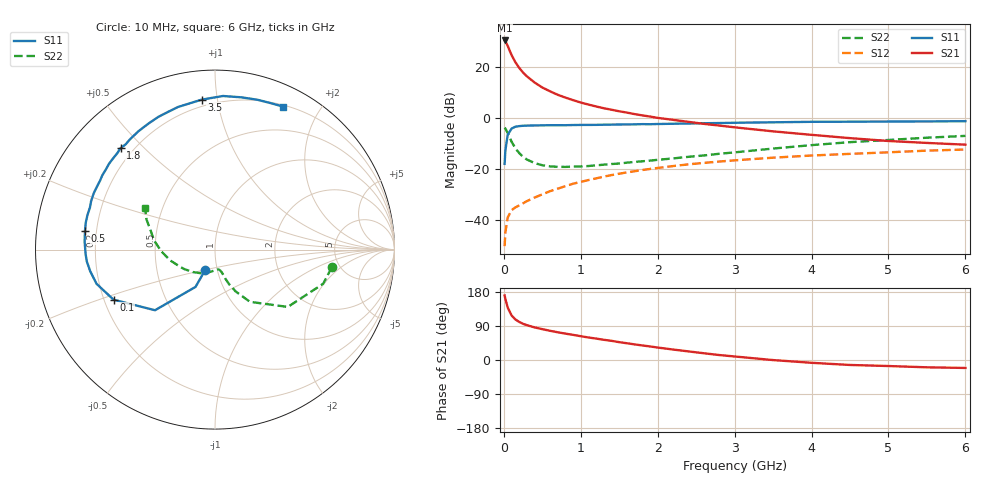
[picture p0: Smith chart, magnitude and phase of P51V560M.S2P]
! SIEMENS Small Signal Semiconductors
! BFP183
! Si NPN RF Bipolar Junction Transistor in SOT143
! VCE = 1.5 V  IC = 60 mA
! Common Emitter S-Parameters:  March  1996
# GHz  S  MA  R  50
!  f  S11  S21  S12  S22
! GHz  MAG  ANG  MAG  ANG  MAG  ANG  MAG  ANG
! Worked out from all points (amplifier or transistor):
!   36 points, 10 MHz to 6 GHz, reference 50 ohm
!   highest |S21| = 30.6 dB at 10 MHz (marker M1)
!   |S21| within 3 dB of that: start of sweep to 62.21 MHz
!   unconditionally stable (mu >= 1): start of sweep to 38.8 MHz; 140 MHz to end of sweep
!   at 250 MHz: K = 1.35, MAG = 22.1 dB, |S12| = -33.4 dB
!   at 1.4 GHz: K = 1.88, MAG = 7.4 dB, |S12| = -22.3 dB
!   at 6 GHz: K = 1.50, MAG = -3.2 dB, |S12| = -12.2 dB
!   S11 on the Smith chart (normalised r, x): 10 MHz: 0.87, -0.20; 100 MHz: 0.24, -0.22; 500 MHz: 0.16, +0.07; 1.8 GHz: 0.15, +0.43; 3.5 GHz: 0.16, +0.90; 6 GHz: 0.22, +1.56
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0.01  0.128 -115.6  33.93 170.4  0.0031 62.5  0.6581 -8.6
0.02  0.2347 -117.6  32.8 161.2  0.0058 63.8  0.6322 -17.5
0.05  0.4754 -134.7  26.58 138.5  0.0113 56.8  0.5165 -38.2
0.1  0.6302 -153.7  17.55 117.8  0.0158 44.8  0.3502 -56.2
0.15  0.687 -163.9  12.7 107.0  0.0179 43.7  0.2592 -63.8
0.2  0.7058 -170.2  9.8 100.4  0.0196 45.9  0.2081 -67.8
0.25  0.7171 -174.7  7.951 95.5  0.0215 47.5  0.1767 -70.0
0.3  0.7213 -177.9  6.697 91.9  0.0238 50.6  0.1557 -71.2
0.4  0.7277 176.5  5.063 86.0  0.0279 54.1  0.1327 -73.4
0.5  0.7317 172.0  4.042 81.4  0.0323 56.4  0.1204 -75.8
0.6  0.7356 168.3  3.406 77.1  0.0372 58.7  0.1144 -78.3
0.7  0.7363 164.8  2.911 73.2  0.0417 59.9  0.1119 -80.6
0.9  0.741 158.7  2.284 66.3  0.0522 60.5  0.1131 -86.2
1.1  0.7453 152.1  1.869 59.4  0.0616 60.6  0.1162 -92.6
1.5  0.7598 141.0  1.38 47.1  0.0821 58.5  0.1301 -105.1
1.8  0.7719 133.0  1.147 38.4  0.0969 55.9  0.1439 -115.5
2.2  0.7856 122.8  0.937 27.6  0.116 51.5  0.1638 -128.4
2.8  0.811 108.6  0.724 13.1  0.1422 44.6  0.2021 -147.3
3.5  0.8388 95.1  0.557 -0.2  0.1694 36.8  0.2559 -166.2
4.5  0.8611 80.1  0.41 -13.1  0.2013 25.5  0.3418 171.7
5.5  0.8728 69.3  0.33 -19.3  0.2331 15.7  0.4179 156.1
6  0.8828 64.5  0.305 -21.0  0.245 10.4  0.4534 149.2
